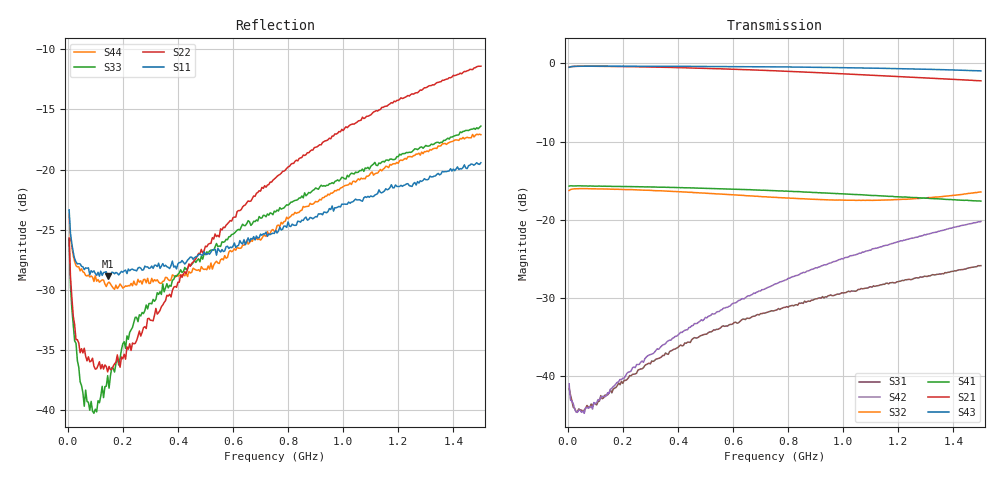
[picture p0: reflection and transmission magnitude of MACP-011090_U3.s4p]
!Agilent Technologies,E5071C,MY46110647,A.11.31
!Date: Tue Jan 18 13:59:39 2022 DD
!Data & Calibration Information:
!MACP-011090 soldered onto PT-0003645 with F connectors, Port1 (pin1) Port2 (pin6) Port3 (pin4) Port4 (pin3)
!Freq	S11:SOLT4(ON)	S12:SOLT4(ON)	S13:SOLT4(ON)	S14:SOLT4(ON)
!	S21:SOLT4(ON)	S22:SOLT4(ON)	S23:SOLT4(ON)	S24:SOLT4(ON)
!	S31:SOLT4(ON)	S32:SOLT4(ON)	S33:SOLT4(ON)	S34:SOLT4(ON)
!	S41:SOLT4(ON)	S42:SOLT4(ON)	S43:SOLT4(ON)	S44:SOLT4(ON)
!PortZ  Port1:75+j0  Port2:75+j0  Port3:75+j0  Port4:75+j0
!Above PortZ is port z conversion or system Z0 setting when saving the data.
!When reading, reference impedance value at option line is always used.
# Hz S MA R 75
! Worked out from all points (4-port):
!   300 points, 5 MHz to 1.5 GHz, reference 75 ohm
!   strongest paths, dB at 5 MHz, 380 MHz, 755 MHz, 1.13 GHz, 1.5 GHz:
!     S43: -0.5, -0.4, -0.4, -0.6, -0.9
!     S21: -0.5, -0.5, -0.9, -1.5, -2.2
!     S41: -15.7, -15.9, -16.3, -16.9, -17.6
!     S32: -16.3, -16.4, -17.1, -17.5, -16.5
!     S42: -41.0, -35.2, -28.2, -23.5, -20.2
!     S31: -41.6, -36.7, -31.6, -28.4, -25.9
!   lowest |S11| = -28.9 dB at 145 MHz (marker M1), VSWR 1.07, Z = 70.4 + j2.51 ohm
!   |S11| at or under -10 dB: start of sweep to end of sweep
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5000000  0.06804 145.8  0.9477 2.1  0.009513 139.6  0.1641 179.8
         0.9471 2.1  0.05194 127.2  0.154 4.9  0.008567 143.8
         0.00831 146.2  0.1537 4.2  0.05152 123.3  0.9466 2.3
         0.1641 -179.9  0.008891 141.5  0.9461 2.3  0.06509 142.9
3e7  0.04135 156.2  0.9594 -0.6  0.005693 152.6  0.1645 177.4
     0.9594 -0.6  0.01965 137.8  0.1578 0.6  0.005993 172.1
     0.005904 150.1  0.1577 0.7  0.01897 142.0  0.9593 -0.2
     0.1645 177.3  0.00587 174.2  0.9597 -0.2  0.03988 163.0
6e7  0.03842 159.7  0.9613 -2.1  0.006042 145.7  0.1642 174.6
     0.9605 -2.1  0.0181 130.1  0.1581 -0.4  0.006438 -173.4
     0.006027 144.8  0.158 -0.4  0.01039 160.2  0.961 -1.4
     0.1643 174.6  0.005754 -172.5  0.9609 -1.4  0.03731 172.3
1.45e8  0.03605 150.3  0.9585 -5.8  0.007377 121.5  0.1636 167.0
        0.9582 -5.8  0.01443 112.8  0.157 -2.1  0.008014 -160.0
        0.007553 124.7  0.1571 -2.1  0.01392 -141.4  0.9612 -4.1
        0.1636 167.0  0.007799 -160.0  0.9609 -4.1  0.03368 -174.4
3.45e8  0.04065 116.9  0.946 -13.9  0.01344 87.0  0.1614 149.5
        0.9458 -13.9  0.02737 47.5  0.1527 -4.9  0.0153 -166.7
        0.01351 90.7  0.1528 -5.0  0.0335 -109.3  0.9588 -10.0
        0.1613 149.5  0.01579 -167.2  0.9591 -10.1  0.03428 -149.5
6.35e8  0.04907 72.2  0.9145 -25.1  0.02293 61.2  0.1564 124.5
        0.914 -25.1  0.07001 1.9  0.1432 -6.6  0.03059 163.8
        0.02305 64.0  0.1432 -6.7  0.05931 -105.0  0.9546 -18.7
        0.1561 124.3  0.03123 163.8  0.9548 -18.7  0.04859 -122.6
1.5e9  0.1068 -26.3  0.7752 -55.0  0.0505 9.3  0.1323 51.3
       0.7742 -55.0  0.2692 -70.1  0.1525 6.9  0.09456 75.4
       0.05075 12.3  0.1505 6.5  0.1517 -101.3  0.8956 -46.6
       0.1314 51.7  0.09736 76.5  0.8969 -46.6  0.1398 -121.1
